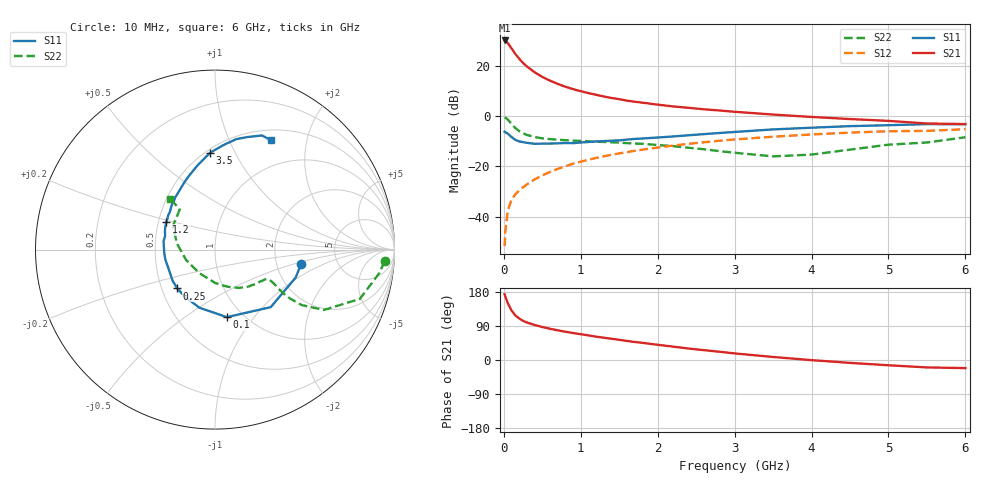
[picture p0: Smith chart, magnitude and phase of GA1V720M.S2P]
! Infineon Technologies  Discrete & RF Semiconductors
! BF775
! Si NPN RF Bipolar Junction Transistor in SOT23
! VCE = 1.75 V  IC = 20 mA
! Common Emitter S-Parameters:  May  1996
# GHz  S  MA  R  50
!  f  S11  S21  S12  S22
! GHz  MAG  ANG  MAG  ANG  MAG  ANG  MAG  ANG
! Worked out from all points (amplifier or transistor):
!   36 points, 10 MHz to 6 GHz, reference 50 ohm
!   highest |S21| = 30.0 dB at 10 MHz (marker M1)
!   |S21| within 3 dB of that: start of sweep to 96.55 MHz
!   unconditionally stable (mu >= 1): 308.9 MHz to 4.202 GHz; 5.105 GHz to end of sweep
!   at 250 MHz: K = 0.93, MSG = 24.7 dB, |S12| = -28.3 dB
!   at 1.4 GHz: K = 1.16, MAG = 8.9 dB, |S12| = -15.4 dB
!   at 6 GHz: K = 1.01, MAG = 0.4 dB, |S12| = -5.3 dB
!   S11 on the Smith chart (normalised r, x): 10 MHz: 2.75, -0.59; 100 MHz: 0.84, -0.74; 250 MHz: 0.60, -0.29; 1.2 GHz: 0.55, +0.19; 3.5 GHz: 0.53, +0.80; 6 GHz: 0.63, +1.44
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0.01  0.4862 -9.7  31.52 173.6  0.0026 83.3  0.947 -3.9
0.02  0.4757 -19.1  31.04 167.2  0.0052 81.6  0.9251 -8.1
0.05  0.4464 -45.9  28.25 150.6  0.013 73.9  0.8525 -18.8
0.1  0.3821 -80.0  21.93 130.6  0.0217 66.7  0.6937 -29.0
0.15  0.3353 -104.9  16.97 117.5  0.0279 64.3  0.5735 -32.6
0.2  0.3124 -121.6  13.66 109.4  0.0332 64.7  0.5001 -33.1
0.25  0.302 -134.3  11.26 103.4  0.0385 65.1  0.4519 -32.6
0.3  0.2927 -143.8  9.58 98.9  0.0437 66.9  0.4195 -31.7
0.4  0.2799 -158.0  7.37 92.5  0.055 68.0  0.3816 -30.1
0.5  0.2822 -168.7  5.956 87.0  0.066 68.8  0.3593 -29.3
0.6  0.2834 -176.7  5.018 82.4  0.0775 69.1  0.3465 -29.1
0.7  0.2856 176.4  4.332 78.3  0.0887 69.1  0.3378 -29.4
0.8  0.2903 170.8  3.805 74.6  0.1005 68.2  0.3301 -30.0
0.9  0.2882 164.7  3.408 71.2  0.1125 68.0  0.3235 -30.8
1.1  0.304 155.7  2.842 64.9  0.135 66.4  0.3142 -33.8
1.2  0.3122 150.3  2.629 61.6  0.1466 65.4  0.3084 -35.2
1.6  0.3392 136.2  2.015 50.2  0.1918 60.9  0.2887 -42.9
2.2  0.3916 119.1  1.545 35.3  0.258 53.6  0.2515 -58.0
3.5  0.5403 92.9  1.066 8.0  0.387 35.5  0.1576 -122.7
4.5  0.6275 79.0  0.868 -7.6  0.467 21.3  0.2146 171.0
5.5  0.6878 67.6  0.708 -19.6  0.5061 6.7  0.2973 131.4
6  0.6846 63.0  0.69 -21.4  0.5458 2.6  0.3776 131.2
